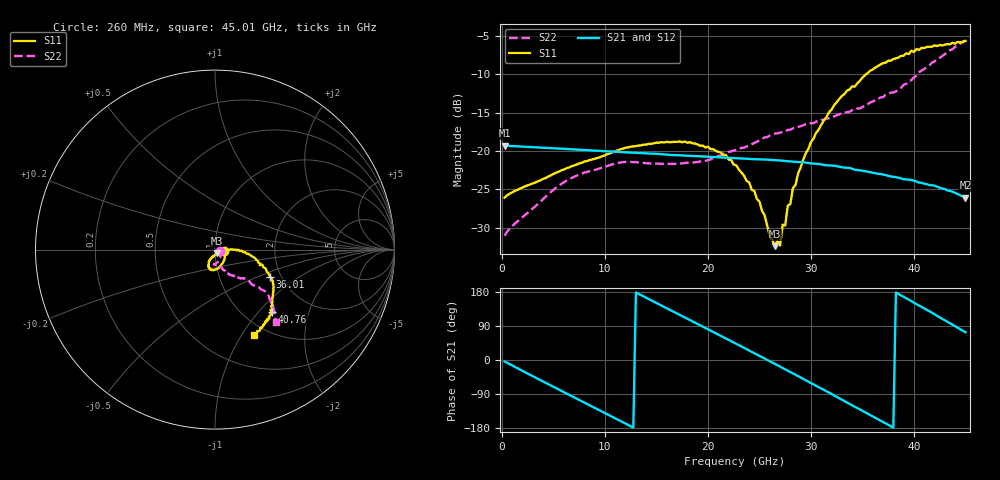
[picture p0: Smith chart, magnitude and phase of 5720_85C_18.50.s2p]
! Device:  ADRF5720
! Description: 0.5dB LSB GaAs MMIC 6-bit Digital Attenuator
! Frequency:  0.000009 -  40 GHz
! Ports:
!	RF1	= Port 1
!	RF2	= Port 2
! Vdd:  3.3 Volt
! Vss:  -3.3 Volt
! Control:  0/3.3 Volt
! State:  18.50 dB attenuation
! Data:  The device was measured using G-S-G Probes on a matrix board.
!  Data was collected using an calibrated 4 port network analyzer.
!  The reference plane for this measurement is at the launchers.
! Note:  Analog Devices supplies this data as a sample of measured data
!  for this product.  Your particular data for this product may vary.
!  Data was taken at 85 degrees C.
!  Analog Devices reserves the right to change this data at anytime.
# GHZ S DB R 45.0
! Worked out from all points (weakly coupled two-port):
!   180 points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, 260 MHz to 45.01 GHz, reference 45 ohm
!   highest |S21| = -19.28 dB at 260 MHz (marker M1); lowest = -26.1 dB at 45.01 GHz (marker M2)
!   lowest |S11| = -32.4 dB at 26.51 GHz (marker M3), VSWR 1.05, Z = 45.9 - j1.99 ohm
!   |S11| at or under -10 dB: start of sweep to 35.35 GHz
!   |S22| runs from -31.1 to -5.6 dB; largest |S21 - S12| = 0.00052
!   S11 on the Smith chart (normalised r, x): 260 MHz: 1.10, -0.02; 36.01 GHz: 1.75, -0.60; 40.76 GHz: 1.32, -1.19; 45.01 GHz: 0.87, -1.14
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0.26  -26.08 -10.4  -19.28 -3.9  -19.28 -3.9  -31.05 -17.4
5.01  -22.98 -39.9  -19.64 -70.9  -19.62 -70.8  -25.05 -61.5
7.76  -21.54 -57.3  -19.84 -109.1  -19.83 -109.0  -22.94 -78.0
11.51  -19.77 -77.2  -20.13 -160.9  -20.12 -160.8  -21.49 -91.9
15.26  -18.91 -92.6  -20.39 146.9  -20.37 147.0  -21.65 -93.9
20.01  -19.43 -108.7  -20.74 80.9  -20.72 81.1  -21.18 -80.4
22.76  -21.86 -114.3  -20.94 42.6  -20.92 42.8  -19.85 -72.1
25.01  -26.59 -108.4  -21.08 11.1  -21.06 11.3  -18.58 -68.8
26.51  -32.42 -64.7  -21.19 -10.3  -21.18 -10.1  -17.72 -65.2
26.76  -31.69 -51.3  -21.21 -13.9  -21.19 -13.7  -17.68 -65.1
27.01  -32.36 -36.8  -21.23 -17.6  -21.21 -17.3  -17.60 -64.2
27.26  -29.62 -24.8  -21.27 -21.2  -21.25 -20.9  -17.50 -64.5
27.51  -29.71 -16.0  -21.30 -24.7  -21.29 -24.4  -17.44 -63.5
27.76  -27.12 -11.1  -21.33 -28.3  -21.31 -28.0  -17.25 -64.1
28.01  -26.91 -8.1  -21.36 -31.9  -21.35 -31.6  -17.21 -63.4
28.26  -24.83 -4.7  -21.39 -35.4  -21.37 -35.1  -17.04 -63.8
30.26  -18.38 -2.2  -21.63 -64.3  -21.62 -64.0  -16.37 -61.3
33.01  -12.80 -12.2  -22.12 -104.7  -22.10 -104.5  -15.07 -55.8
36.01  -9.35 -26.2  -22.83 -148.9  -22.80 -148.6  -13.54 -49.1
37.76  -8.20 -33.5  -23.32 -174.8  -23.30 -174.4  -12.38 -43.6
40.76  -6.52 -47.7  -24.15 140.0  -24.12 140.4  -9.48 -40.9
45.01  -5.63 -65.2  -26.07 73.3  -26.05 73.6  -5.56 -50.1
